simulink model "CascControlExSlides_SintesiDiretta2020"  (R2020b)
settings: Solver=ode4  StartTime=0.0  StopTime=100  FixedStep=0.001  RelTol=1e-3
undefined symbols (not defined in the file or in its folder): dR, dR1, dR2, nR, nR1, nR2

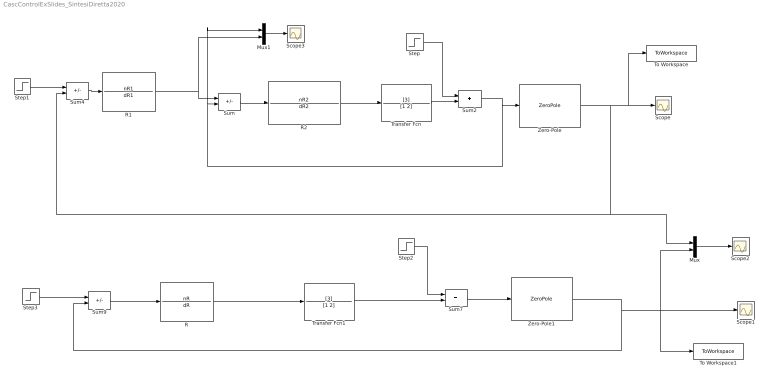
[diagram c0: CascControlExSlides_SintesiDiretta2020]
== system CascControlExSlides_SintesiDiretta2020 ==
  Mux : Mux  Inputs=2
  Mux1 : Mux  Inputs=2
  R : TransferFcn  Numerator=nR  Denominator=dR
  R1 : TransferFcn  Numerator=nR1  Denominator=dR1
  R2 : TransferFcn  Numerator=nR2  Denominator=dR2
  Scope{,1..3} (4 alike) : Scope
  Step : Step  Time=50  SampleTime=0
  Step1 : Step  Time=0  SampleTime=0
  Step2 : Step  Time=50  SampleTime=0
  Step3 : Step  Time=0  SampleTime=0
  Sum : Sum  Inputs=+-
  Sum2 : Sum
  Sum4 : Sum  Inputs=+-
  Sum7 : Sum
  Sum9 : Sum  Inputs=+-
  To Workspace : ToWorkspace  VariableName=ycasc  SaveFormat=Timeseries  SampleTime=-1
  To Workspace1 : ToWorkspace  VariableName=ysl  SaveFormat=Timeseries  SampleTime=-1
  Transfer Fcn : TransferFcn  Numerator=[3]  Denominator=[1 2]
  Transfer Fcn1 : TransferFcn  Numerator=[3]  Denominator=[1 2]
  Zero-Pole : ZeroPole  Zeros=[]  Poles=[-1 -1 -1]  Gain=10
  Zero-Pole1 : ZeroPole  Zeros=[]  Poles=[-1 -1 -1]  Gain=10
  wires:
  R2/1 -> Transfer Fcn/1
  Transfer Fcn/1 -> Sum2/2
  Sum2/1 -> Zero-Pole/1, Mux1/1, Sum/2
  Step/1 -> Sum2/1
  R1/1 -> Sum/1, Mux1/2
  Zero-Pole/1 -> To Workspace/1, Scope/1, Mux/1, Sum4/2
  Step1/1 -> Sum4/1
  Step3/1 -> Sum9/1
  Zero-Pole1/1 -> To Workspace1/1, Mux/2, Scope1/1, Sum9/2
  Step2/1 -> Sum7/1
  Sum7/1 -> Zero-Pole1/1
  Transfer Fcn1/1 -> Sum7/2
  Mux/1 -> Scope2/1
  Sum/1 -> R2/1
  Mux1/1 -> Scope3/1
  Sum4/1 -> R1/1
  Sum9/1 -> R/1
  R/1 -> Transfer Fcn1/1
